PROGRAM vision
VAR
	// 系统变量，控制程序步
	State						:	CurrentState := CurrentState.Init;
	// 初始化工作步
	stepinit					:	INT := 0;
	// 载入轮廓工作步
	stepload					:	INT := 0;
	// 配方触发器
	readtrig					:	r_trig;
	// 外部触发视觉提交
	VisionTrig					:	R_TRIG;
	// 配方相关
	bReadRecipe					:	BOOL;
	// 循环/计数变量
	i							:	ULINT;
	j							:	ULINT;
	l							:	ULINT;
	m							:	DINT;
	// 视觉变量
	// 视觉系统变量
	hr							:	HRESULT;
	// 颜色
	aColorRed 					: 	TcVnVector4_LREAL := [255, 0, 0];
	aColorGreen 				: 	TcVnVector4_LREAL := [0, 255, 0];	
	aColorBlue 					: 	TcVnVector4_LREAL := [0, 20, 255];
	// 相机
	fbCamera					:	FB_VN_SimpleCameraControl;
	// 相机状态
	eState						:	ETcVnCameraState;
	// 9点标定模式相关变量
	aCircleCenter				:	TcVnPoint2_REAL;
	rCircle						:	REAL;
	aOffsetPoint				:	ARRAY[0..8] OF TcVnPoint2_REAL;
	// 标定点容器
	aSrcPoints					: 	ITcVnContainer;
	aDestPoints 				:  	ITcVnContainer;
	aOffsetPoints 				:  	ITcVnContainer;
	
	// 开启坐标变换
	bTransForm					:	BOOL; // 自动开启
	// 工作步状态信息
	// 轮廓过滤工作信息
	ContourFilterMessage		:	WSTRING;
	// 坐标变换工作信息
	GetMatrixKnMessage			:	WSTRING;
	// 错误信息
	ErrMessage					:	WSTRING;
	// 工作错误状态计时器
	ErrTon						:	ton;
	// 视觉启动延时
	VisionStartDelay			:	ton;
	// 开始工作
	bStart						:	BOOL;
	// 图片以及用于显示的绘制图像
	ipImageIn					:	ITcVnImage;// 相机输入图像
	ipImageInDisp				:	ITcVnDisplayableImage;	
	ipImageWork					:	ITcVnImage;// 工作处理图像
	ipImageWorkDisp				:	ITcVnDisplayableImage;
	ipImageRes					:	ITcVnImage;// 处理结果
	ipImageResDisp				:	ITcVnDisplayableImage;	// 结果显示窗口
	ipImageBuffer				:	ITcVnImage;// 提取坐标的时刻截取的图像
	ipImageBufferDisp			:	ITcVnDisplayableImage;	// 最近一次拍摄到的物料
	ipImageCalibration			:	ITcVnImage;// 标定坐标点记录
	ipImageCalibrationDisp		:	ITcVnDisplayableImage;
	// 轮廓提取
	// 轮廓
	ipContourList				:	ITcVnContainer;
	ipContour					:	ITcVnContainer;	
	aOffset						:	TcVnPoint;
	// 提取到的轮廓个数
	nNumberOfElements			: 	ULINT;
	// 标定模式二值化阈值
	lrCalibrationThreshold		:	LREAL := 41;
	// 采样模式二值化阈值
	lrCatchThreshold			:	LREAL := 41;
	// 二值化
	// 二值化阈值
	lrThreshold					:	LREAL := 25;
	// 结构元
	ipImageElement				:	ITcVnImage;
	// 结构元类型
	StructuralShape				:	ETcVnStructuringElementShape;
	// 结构元大小
	elementWidth				:	UDINT := 3;
	elementHeight				:	UDINT := 3;
	// 面积过滤
	fArea						:	LREAL;	// 轮廓面积
	// 手动触发视觉计算
	TrigExcute					:	BOOL := FALSE;
	// 捕获视野中的标定点坐标
	bstartGetData				:	BOOL := FALSE;
	// 刷新标定点坐标，用于标定，更新视觉中的标定点组
	bRefreshData				:	BOOL := FALSE; // 视觉9点提取
	// 手动转换
	ManualChange				:	BOOL;
	// 强制提交数据
	ForcePush					:	BOOL := FALSE;
	// 面积过滤阈值下限，用于轮廓提取
	fAreaMin					:	LREAL := 45000; // 实际面积最小值
	// 标定图形面积过滤上下限，依据标定图纸确定，需要配合专用标定纸使用
	calibrationMin				:	LREAL := 8000;
	calibrationMax				:	LREAL := 40000;
	// 坐标提取
	aCenter						:	TcVnPoint2_LREAL; // 质心坐标
	aCenterActPos				:	TcVnPoint2_LREAL; // 输出物料抓取点像素坐标
	stRectangle					:	TcVnRotatedRectangle; // 外接矩形坐标
	// 校验点
	aManualPoint				:	TcVnPoint2_LREAL;
	aRobotPoint					:	TcVnPoint2_LREAL;
	// 图片信息变量
	imageinfo					:	TcVnImageInfo;
	imageWidth					:	LREAL;	// 图片宽度（X轴方向）
	imageHeight					:	LREAL;	// 图片高度
	// 拍摄区间
	areaLength					:	LREAL := 0; // 拍摄视野的行程（可能是X或者Y）
	judgePos					:	array[0..1] of LREAL; // 用于判断物体位置的坐标
	areaBuffer					:	LREAL := 50;// 拍摄区间大小
	BeltVelo					:	LREAL := 100; // 皮带运行速度
	// 抓取点坐标
	aCenterPick					:	TcVnPoint2_LREAL; // 抓取点坐标
	// 角度
	Angle						:	LREAL;	// 与X轴（机器人坐标系）夹角（角度制）
//	fAngleTemp					:	LREAL;	// 角度临时变量
	// 缓存（用于去重）
	bmaterialBuffer1				:	DUT_material;
	// 去重坐标阈值（xy）
	xFilter						:	LREAL := 15; // X方向的偏差范围
	yFilter						:	LREAL := 15; // Y方向的偏差范围
	// 物料坐标XY偏移，用于最终调整
	xbias						:	LREAL := 0;
	ybias						:	LREAL := 0;
	// 临时字符串（用于9点标定）
	tempstr: ARRAY[0..8] OF STRING := ['0', '1', '2', '3', '4', '5', '6', '7', '8'];
	// 测量时间
	fbGetCalTime				:	Profiler;
END_VAR

CASE State OF
	CurrentState.Init:
		// 初始化模式
		Step_Init();
	
	CurrentState.Waiting:
		// 等待触发信号模式
		Step_Waiting();
		
	CurrentState.Catchmaterial:
		// 视觉系统开始工作，提取物料
		Step_Catchmaterial();
		
	CurrentState.Calibration:
		// 标定模式，配合特质的标定板，定位坐标
		Step_Calibration();
		

	CurrentState.Error:
		// 出现报错，出现各种错误
		Step_Err();
		
END_CASE

ACTION CameraStartAcquisition:
(*******************************************
切换相机状态到输出图片，复位图片检测变量
*******************************************)

// 切换相机状态
fbCamera.StartAcquisition();
// 未提取到图像
bGetImage := FALSE;
END_ACTION

ACTION ContourFilter:
(*******************************************
轮廓过滤，坐标提取
由相机自行判断中心坐标到达指定区域进行拍摄，提取相应的坐标信息
先通过面积进行粗过滤
然后通过后续的精确过滤提取到物料并做计算
*******************************************)

// 判定轮廓数量多少
IF nNumberOfElements>=1 THEN
	// 提取到至少1个轮廓
	ContourFilterMessage := "已提取到轮廓";
	
	// 重置质心坐标
	aCenter[0]:=0;
	aCenter[1]:=0;
	
	// 遍历轮廓
	FOR i:=0 TO (nNumberOfElements-1) DO
		// 提取面积
		GetContourArea();
		// 面积过滤，对不符合要求（面积特别小）的轮廓直接过滤
		IF fArea> fAreaMin THEN
			
				// 绘制轮廓
				GetAndDrawContour();			
				// 触发坐标提取，去重，信息提交
				GetMaterialMessage();
			
		END_IF		
	END_FOR

ELSE
	bVisionWarning := TRUE;
	ContourFilterMessage := "未提取到至少1个轮廓";
END_IF
END_ACTION

ACTION DrawPic:
(*******************************************
将图像绘制到可见图片，可以使用adsimage watch进行观察
*******************************************)

// 绘制图像
hr := F_VN_TransformIntoDisplayableImage(ipImageIn, ipImageInDisp, S_OK);
hr := F_VN_TransformIntoDisplayableImage(ipImageWork, ipImageWorkDisp, S_OK);		
hr := F_VN_TransformIntoDisplayableImage(ipImageRes, ipImageResDisp, S_OK);
hr := F_VN_TransformIntoDisplayableImage(ipImageBuffer, ipImageBufferDisp, S_OK);
hr := F_VN_TransformIntoDisplayableImage(ipImageCalibration, ipImageCalibrationDisp, S_OK);
END_ACTION

ACTION FindContours:
(*******************************************
轮廓提取
提取二值化后的视野中的所有轮廓
*******************************************)

// 轮廓提取
hr := F_VN_FindContoursExp(
	ipSrcImage:=ipImageWork , 
	ipContours:=ipContourList , 
	eRetrievalMode:=TCVN_CRM_EXTERNAL , 
	eApproximationMethod:=TCVN_CAM_SIMPLE , 
	aOffset:=aOffset , 
	hrPrev:=hr );
// 获取轮廓数量
hr := ipContourList.GetElementNum(nNumberOfElements);
END_ACTION

ACTION GetAndDrawContour:
(*******************************************
绘制轮廓相关信息
提取质心并绘制
提取外接矩形并绘制
提取外界矩形的几何中心并绘制
*******************************************)

// 面积满足条件
ContourFilterMessage := "已提取到面积符合的对象";
// 取得质心
hr := F_VN_ContourCenterOfMass(ipContour , aCenter, hr );
// 外接矩形
hr := F_VN_EnclosingRectangle(ipContour , stRectangle , hr );
// 在工作区域图片上绘制轮廓（绿色）
hr := F_VN_DrawContours(
		ipContours:=ipContour , 
		nContourIndex:=-1 , 
		ipDestImage:=ipImageRes , 
		aColor:=aColorGreen , 
		nThickness:=2 , 
		hrPrev:=hr );
// 在工作区域图片上绘制质心（绿色）
hr := F_VN_DrawPointExp(
		nX:=TO_UDINT(aCenter[0]), 
		nY:=TO_UDINT(aCenter[1]), 
		ipDestImage:=ipImageRes , 
		eShape:=TCVN_DS_PLUS , 
		aColor:=aColorGreen , 
		nSize:=10 , 
		nThickness:=3 , 
		eLineType:=TCVN_LT_8_CONNECTED , 
		hrPrev:=hr );
// 在工作区域图片上绘制矩形框（红色）
hr := F_VN_DrawRotatedRectangle(
		stRectangle:= stRectangle, 
		ipDestImage:= ipImageRes, 
		aColor:= aColorRed, 
		nThickness:= 3, 
		hrPrev:= hr);
// 绘制矩形的中心坐标点（红色）
hr := F_VN_DrawPointExp(
		nX:=TO_UDINT(stRectangle.aCenter[0]), 
		nY:=TO_UDINT(stRectangle.aCenter[1]), 
		ipDestImage:=ipImageRes , 
		eShape:=TCVN_DS_PLUS , 
		aColor:=aColorRed , 
		nSize:=10 , 
		nThickness:=3 , 
		eLineType:=TCVN_LT_8_CONNECTED , 
		hrPrev:=hr );
END_ACTION

ACTION GetCalibrationPoint:
(*******************************************
使用轮廓提取的方式，获取标定点坐标
*******************************************)

// 判定轮廓数量多少
IF nNumberOfElements>=1 AND bstartGetData THEN
	// 提取到至少1个轮廓
	// 遍历轮廓
	j := 0;
	FOR i:=0 TO (nNumberOfElements-1) DO
		// 提取到具体轮廓
		hr := F_VN_GetAt_ITcVnContainer(ipContourList ,ipContour , i , hr );
		// 提取轮廓面积
		hr := F_VN_ContourArea(ipContour , fArea, hr );
		// 面积过滤
		IF (fArea > calibrationMin) AND (fArea < calibrationMax) THEN;
			// 面积满足条件
			// 外接圆（圆心坐标为相对于提取区域的坐标）
			hr := F_VN_EnclosingCircle(ipPointSet:= ipContour, aCenter:= aCircleCenter, fRadius:= rCircle, hrPrev:= hr);
			hr := F_VN_EnclosingRectangle(ipContour , stRectangle , hr );
			// 绘制标定圆心
			hr := F_VN_DrawPointExp(
					nX:=TO_UDINT(aCircleCenter[0]), 
					nY:=TO_UDINT(aCircleCenter[1]), 
					ipDestImage:=ipImageRes , 
					eShape:=TCVN_DS_PLUS , 
					aColor:=aColorGreen , 
					nSize:=10 , 
					nThickness:=3 , 
					eLineType:=TCVN_LT_8_CONNECTED , 
					hrPrev:=hr );
			// 提取到的坐标注入数组
			IF j <= 8 THEN
				// 绘制点号
				hr := F_VN_PutTextExp(
					sText:= tempstr[j], 
					ipDestImage:= ipImageRes, 
					nX:= TO_UDINT(aCircleCenter[0]+25), 
					nY:= TO_UDINT(aCircleCenter[1] + 25), 
					eFontType:= ETcVnFontType.TCVN_FT_HERSHEY_PLAIN, 
					fFontScale:= 10, 
					aColor:= aColorRed, 
					nThickness:= 4, 
					eLineType:= 4, 
					bBottomLeftOrigin:= FALSE, 
					hrPrev:= hr);
				// 更新视觉矩阵数组
				IF bRefreshData THEN
					aSrcPoint[j][0] := aCircleCenter[0];
					aSrcPoint[j][1]	:= aCircleCenter[1];
				END_IF
				j := j+ 1;
			END_IF
			IF bRefreshData THEN
				hr := F_VN_CopyImageRegion(
					ipSrcImage:= ipImageRes, 
					nX:= 0, 
					nY:= 0, 
					nWidth:= imageinfo.nWidth, 
					nHeight:= imageinfo.nHeight, 
					ipDestImage:= ipImageCalibration, 
					hrPrev:= hr);
			END_IF
		END_IF
	END_FOR
END_IF
END_ACTION

ACTION GetContourArea:
(*******************************************
轮廓面积提取
对于轮廓进行面积计算
*******************************************)

// 有轮廓
bVisionWarning := FALSE;
// 提取到具体轮廓
hr := F_VN_GetAt_ITcVnContainer(ipContourList ,ipContour , i , hr );
// 提取轮廓面积
hr := F_VN_ContourArea(ipContour , fArea, hr );
END_ACTION

ACTION GetdMaterial:
(*******************************************
数据注入结构体
*******************************************)

// 注入机器人结构体
dMaterial.bMaterial := TRUE;
// 机器人需要旋转的角度为机器人坐标正向90度
IF Angle < 90 THEN
	dMaterial.lrAngle :=  (Angle);
ELSE
	dMaterial.lrAngle := -(90 - Angle);
END_IF
//dMaterial.lrAngle := Angle;
// 提取点坐标注入
dMaterial.lrCenterX := aCenterActPos[0] + xbias;// 坐标偏置
dMaterial.lrCenterY := aCenterActPos[1] + ybias;
// 输出面积
dMaterial.lrArea := fArea;	
// 拍摄图片的时间（获取系统时间求得）
dMaterial.lrPhotoTime := ULINT_TO_LREAL(F_GetSystemTime()) / 10000000;
dMaterial.lrPhotoBeltPos:=BeltAxis.NcToPlc.ActPos;
END_ACTION

ACTION GetImageWH:
(*******************************************
读取图片信息，主要是获取宽度值
*******************************************)

// 读取相机输入图像信息
hr := F_VN_GetImageInfo(ipImage:= ipImageIn, stImageInfo:= imageinfo, hrPrev:= hr);

// 将信息提取到指定变量
imageWidth := TO_LREAL(imageinfo.nWidth);
imageHeight := TO_LREAL(imageinfo.nHeight);
END_ACTION

ACTION GetMaterialMessage:
(*******************************************
拍摄
计算指定区间
判断外接矩形的中心坐标是否达到指定区域
如果到达指定区域，则对物料做后续计算以及坐标提取
*******************************************)


// 手动触发器，如果触发，则强制拍摄
VisionTrig(CLK:= TrigExcute, Q=> );
// 使用X判断/Y判断，皮带的X方向与相机的X方向/Y方向重合，建议不要使用，需要修改后续的逻辑
	areaLength := imageHeight / 2;
	judgePos[0] := stRectangle.aCenter[1];
	judgePos[1] := stRectangle.aCenter[0];
// 判断外接矩形的中心点是否在指定区域或强制推送
IF (judgePos[0] > areaLength - areaBuffer) AND (judgePos[0] < areaLength + areaBuffer) AND (judgePos[1] > 200) AND (judgePos[1] < (imageWidth - 200)) 
	OR VisionTrig.Q OR ForcePush THEN
	// 通过矩形的角度求得实际物体的部署角度
	Angle := TO_LREAL(stRectangle.fAngle);
	
	// 提取点坐标，提取点坐标为质心坐标
		aCenterPick[0] := aCenter[0];
		aCenterPick[1] := aCenter[1];
		
	
	
	// 绘制提取点
	hr := F_VN_DrawPointExp(
		nX:=TO_UDINT(aCenterPick[0]), 
		nY:=TO_UDINT(aCenterPick[1]), 
		ipDestImage:=ipImageRes , 
		eShape:=TCVN_DS_PLUS , 
		aColor:=aColorBlue , 
		nSize:=10 , 
		nThickness:=3 , 
		eLineType:=TCVN_LT_8_CONNECTED , 
		hrPrev:=hr );
		
	// 结果注入队列
	PushbMaterial();
END_IF
END_ACTION

ACTION GetTransformationMatrixKn:
(*******************************************
生成变换矩阵
将变换矩阵用的点位（视觉坐标系9点，机器人坐标系9点），分别注入container
通过2个container求解变换矩阵
*******************************************)

// 坐标变换
FOR j := 0 TO 8 BY 1 DO
	// 机器人坐标系标定时需要减去皮带偏移，相机不在机器人正下方
	aOffsetPoint[j][0] := aDestPoint[j][0] - lrBeltOffset;
	aOffsetPoint[j][1] := aDestPoint[j][1];
END_FOR

// 生成变换点集
hr := F_VN_CreateContainerFromArray(
	pData:= ADR(aSrcPoint), 
	ipContainer:= aSrcPoints, 
	nTypeGuid:= ContainerType_Vector_TcVnPoint2_REAL, 
	nElementNum:= 9, 
	hrPrev:= 0);// 视觉像素点集
hr := F_VN_CreateContainerFromArray(
	pData:= ADR(aOffsetPoint), 
	ipContainer:= aOffsetPoints, 
	nTypeGuid:= ContainerType_Vector_TcVnPoint2_REAL, 
	nElementNum:= 9, 
	hrPrev:= 0);// 机器人坐标系点集

// 判断点集合是否有效（如果没有成功上载配方，点集可能是无效的，将会触发pagefault）
IF (aSrcPoints <> 0) AND (aOffsetPoints <> 0) THEN
	// 获取变换矩阵
	hr := F_VN_Homography(aSrcPoints, aOffsetPoints, aTransformationMatrix, 0);
	// 坐标变换矩阵求解成功，开启坐标变换
	bTransForm := TRUE;
	GetMatrixKnMessage := "";
ELSE
	// 点集合无效，报错
	bVisionWarning := TRUE;
	bTransForm := FALSE;
	GetMatrixKnMessage := "无效坐标点或变换矩阵";
END_IF


// 释放
FW_SafeRelease(ADR(aSrcPoints));
FW_SafeRelease(ADR(aDestPoints));
END_ACTION

ACTION Halt:
(*******************************************
如果触发了停止信号，就将状态机切换到Waiting状态
*******************************************)

// 触发停止动作
IF VisionHalt THEN
	// 切换到等待状态
	State := CurrentState.Waiting;
	// 对停止信号进行复位操作
	VisionHalt := FALSE;
END_IF
END_ACTION

ACTION Pretreatment:
(*******************************************
预处理
将输入图像转换为三通道图像注入结果图像（方便后续绘制轮廓等）
将输入图像进行二值化，注入工作图像，用于后续计算
*******************************************)

// 单通道变为三通道(RGB)注入结果图像
hr := F_VN_ConvertColorSpace(ipImageIn ,ipImageRes , TCVN_CST_GRAY_TO_RGB , hr );
// 二值化
hr := F_VN_Threshold(
	ipSrcImage:=ipImageIn , 
	ipDestImage:=ipImageWork , 
	fThreshold:=lrThreshold , 
	fMaxValue:=255 , 
	eThresholdType:=TCVN_TT_BINARY , 
	hrPrev:=hr );
END_ACTION

ACTION PushbMaterial:
(*******************************************
坐标变换，去重，提交数据
去重的思路为，物料X坐标以及Y坐标是否一致，一致的话就认为是同一个
对于目前的情况，X坐标还需要减去两次拍摄之间皮带的偏移量
*******************************************)

IF bTransForm THEN
	// 将中心坐标使用变换矩阵转换为机器人坐标系
	hr := F_VN_WarpPerspective_Point(aCenterPick ,aCenterActPos , aTransformationMatrix , hr );
	// 本次拍摄结果坐标与上一次拍摄结果坐标比对进行去重计算，计算xy坐标是否相近，相近则判断为同一个，不做提交
	IF (ABS(bMaterialBuffer1.lrCenterY - aCenterActPos[1]) > YFilter) OR 
	(ABS(ABS(bMaterialBuffer1.lrCenterX - aCenterActPos[0]) - ABS(bMaterialBuffer1.lrPhotoBeltPos - beltAxis.NcToPlc.ActPos)) > YFilter) THEN
			// 注入结构体
			GetdMaterial();
			
			// 绘制提取点
			hr := F_VN_DrawPointExp(
					nX:=TO_UDINT(aCenterPick[0]), 
					nY:=TO_UDINT(aCenterPick[1]), 
					ipDestImage:=ipImageRes , 
					eShape:=TCVN_DS_PLUS , 
					aColor:=aColorBlue , 
					nSize:=10 , 
					nThickness:=3 , 
					eLineType:=TCVN_LT_8_CONNECTED , 
					hrPrev:=hr );
			
			
				// 压入队列
				gfbPushPopStack(ArrayStmaterial:=gArrayStmaterial , PushStmaterial:=dmaterial , PopStmaterial=> , busy=>gbPushPopBusy );
				gfbPushPopStack.PushStack();
				fbGetCalTime(START:= FALSE, RESET:= FALSE, BUSY=> , DATA=> );			
			// 将最后一个写入队列的dmaterial设置为比较对象
			MEMCPY(destAddr:= ADR(bMaterialBuffer1), srcAddr:= ADR(dMaterial), n:= SIZEOF(bMaterialBuffer1));
		
			// 记录拍摄瞬间的时刻的图像
			hr := F_VN_CopyImage(ipSrcImage:= ipImageRes, ipDestImage:= ipImageBuffer, hrPrev:= hr);
	END_IF
END_IF
END_ACTION

ACTION RecipeSaveAndRead:
(*******************************************
配方操作
通过设置好的配方名称，对配方进行读
由于配方主要用于矩阵的保存以及读取，而TwinCAT的配方无法直接保存TcVnPoint2_LREAL型的视觉点变量，因此要先转换为普通的二维数组点
*******************************************)


// 读取配方触发器
readtrig(CLK:= bReadRecipe , Q=> );

// 触发器触发
IF  readtrig.Q THEN
		// 触发读取配方，将配方点数组读取后，写入视觉矩阵
	FOR l := 0 TO 8 BY 1 DO
		aSrcPoint[l][0] := srcpoint[l, 0];
		aSrcPoint[l][1] := srcpoint[l, 1];
		aDestPoint[l][0] := destpoint[l, 0];
		aDestPoint[l][1] := destpoint[l, 1];
	END_FOR
END_IF
END_ACTION

ACTION Release:
(*******************************************
释放内存
*******************************************)

FW_SafeRelease(ADR(ipContourList));
FW_SafeRelease(ADR(ipContour));
END_ACTION

ACTION Step_Calibration:
(*******************************************
标定模式
用于更新参数
将视觉坐标系以及机器人坐标系进行对应
*******************************************)

// 读取相机状态
eState := fbCamera.GetState();

// 相机停止状态监控
Halt();

// 根据状态进行操作
CASE eState OF
// 相机初始化
TCVN_CS_INITIAL,TCVN_CS_OPENING,TCVN_CS_OPENED,TCVN_CS_STARTACQUISITION:
	// 切换相机状态
	CameraStartAcquisition();

TCVN_CS_ACQUIRING:
	// 复位错误计时器
	ErrTon.IN := FALSE;
	// 获取图片
	hr := fbCamera.GetCurrentImage(ipImageIn);
	// 图片采样成功
	IF tc3_module.SUCCEEDED(hr) AND ipImageIn <> 0 THEN
		// 图片提取成功
		bGetImage := TRUE;
		
		// 修改二值化阈值
		lrThreshold := lrCalibrationThreshold;
		
		// 预处理
		Pretreatment();
		
		// 像素取反（标定用的纸为白底黑色圆，需要前景背景替换）
		hr := F_VN_BitwiseNotImage(ipSrcImage:= ipImageWork, ipDestImage:= ipImageWork, hrPrev:= hr);
		// 闭运算
		hr := F_VN_CreateStructuringElement(
			ipStructuringElement:= ipImageElement, 
			eShape:= StructuralShape, 
			nWidth:= elementWidth, 
			nHeight:= elementHeight, 
			hrPrev:= hr);
		hr := F_VN_MorphologicalOperator(
			ipSrcImage:= ipImageWork, 
			ipDestImage:= ipImageWork, 
			eOperator:= TCVN_MO_CLOSING, 
			ipStructuringElement:= ipImageElement, 
			hrPrev:= hr);
		
		// 轮廓提取
		FindContours();
		
		// 获取坐标点
		GetCalibrationPoint();
		
		// 更新坐标变换矩阵
		GetTransformationMatrixKn();
		
		// 校验标定
		IF ManualChange THEN
			// 手动转换，将视觉坐标转换成机器人坐标
			hr := F_VN_WarpPerspective_Point(aManualPoint ,aRobotPoint , aTransformationMatrix , hr );
		END_IF
		
		// 坐标保存(暂时未研究如何配合hmi的recipe)
	//	RecipeSaveAndRead();
		
		// 绘制图像
		DrawPic();

	ELSE
		// 未提取到图像
		bGetImage := FALSE;
	END_IF

Tc3_Vision.TCVN_CS_ERROR:
	// 执行报错动作
	VisionError();
END_CASE
END_ACTION

ACTION Step_Catchmaterial:
(*******************************************
拍摄
正常工作状态
相机无限制拍摄图片，根据拍摄出的图片进行相应的坐标计算，并返还结果
*******************************************)

// 读取相机状态
eState := fbCamera.GetState();

// 相机停止状态监控
Halt();

// 根据状态进行操作
CASE eState OF
// 相机初始化
TCVN_CS_INITIAL,TCVN_CS_OPENING,TCVN_CS_OPENED,TCVN_CS_STARTACQUISITION:
	// 切换相机状态
	CameraStartAcquisition();
	
TCVN_CS_ACQUIRING:
	// 复位错误计时器
	ErrTon.IN := FALSE;
	// 获取图片
	hr := fbCamera.GetCurrentImage(ipImageIn);
	// 图片采样成功
	IF tc3_module.SUCCEEDED(hr) AND ipImageIn <> 0 THEN
		// 图片提取成功
		bGetImage := TRUE;
		
		// 计算时间
//		fbGetCalTime(START:= FALSE, RESET:= TRUE, BUSY=> , DATA=> );
//		fbGetCalTime(START:= TRUE, RESET:= FALSE, BUSY=> , DATA=> );
		// 重新设置二值化阈值到拍摄模式
		lrThreshold := lrCatchThreshold;
		
		
		// 预处理
		Pretreatment();

		// 轮廓提取
		FindContours();
		
		// 由相机自行判断中心坐标到达指定区域进行拍摄，提取相应的坐标信息
		ContourFilter();
		
		// 释放
		Release();
		
		// 绘制图像
		DrawPic();
		
	ELSE
		// 未提取到图像
		bGetImage := FALSE;
	END_IF
	
Tc3_Vision.TCVN_CS_ERROR:
	// 执行报错动作
	VisionError();
END_CASE
END_ACTION

ACTION Step_Err:
(*******************************************
报错状态，输出错误标志位以及报警信息
*******************************************)

bVisionErr := TRUE;
VisionErrMessage := Tc2_Standard.WCONCAT("视觉系统报错，报错信息：", Errmessage);
END_ACTION

ACTION Step_Init:
(*******************************************
初始步
对参数以及文件目录初始化
生成变换矩阵
检测视觉是否成功采集到图像
获取图像长宽等信息
如果一切正常，则自动切换进入等待模式
*******************************************)

CASE stepinit OF
	
		
	
	
	0:// 上载配方
		// 触发配方读动作
		//bReadRecipe := TRUE;
		// 配方程序
		RecipeSaveAndRead();
		stepinit := 40;
		
	40:// 复位配方程序
		RecipeSaveAndRead();
		bReadRecipe := FALSE;
		stepinit := 50;
		
	50:// 数据准备
		// 更新变换矩阵
		GetTransformationMatrixKn();
		// 复位错误状态
		bVisionErr := FALSE;
		Errmessage := "";
		ErrTon.IN := FALSE;
		stepinit := 60;
		
	60:// 检查是否拍摄到图像
		// 读取相机状态
		eState := fbCamera.GetState();
		
		// 根据状态进行操作
		CASE eState OF
			// 相机初始化
			TCVN_CS_INITIAL,TCVN_CS_OPENING,TCVN_CS_OPENED,TCVN_CS_STARTACQUISITION:
				// 切换相机状态
				CameraStartAcquisition();
				
			// 开始获取照片
			TCVN_CS_ACQUIRING:
				// 复位错误计时器
				ErrTon.IN := FALSE;
				// 获取图片
				hr := fbCamera.GetCurrentImage(ipImageIn);
				// 图片采样成功
				IF tc3_module.SUCCEEDED(hr) AND ipImageIn <> 0 THEN
					// 提取到图像成功
					bGetImage := TRUE;
					// 获取视野的长宽
					GetImageWH();
					// 坐标变换正常激活，图片宽高提取成功
					IF bTransForm AND (imageHeight <> 0) AND (imageHeight <> 0) THEN
						// 延时，告知视觉已经就绪
						VisionStartDelay(IN:= bStart, PT:= T#1S, Q=> VisionReady, ET=> );
						bStart := TRUE;
						// 切换到等待模式
						IF VisionReady THEN
							// 视觉状态通过，切换到下一步
							State := CurrentState.Waiting;
							bStart := FALSE;
						END_IF	
					END_IF
					// 绘制图像
					DrawPic();
				ELSE
					// 未提取到图像
					bGetImage := FALSE;
				END_IF
				
			Tc3_Vision.TCVN_CS_ERROR:
					// 执行报错动作
					VisionError();
		END_CASE
END_CASE
END_ACTION

ACTION Step_Waiting:
(*******************************************
等待模式
等待视觉系统开启信号
开启信号可能由主控程序提供，或者是由调试界面输出
*******************************************)

// 如果允许开启视觉系统
IF VisionStartPush THEN
	// 切换到推送图片
	State := CurrentState.Catchmaterial;
	// 对开启信号进行复位操作
	VisionStartPush := FALSE;
END_IF
END_ACTION

ACTION VisionError:
(*******************************************
相机出现报错，检测报错能否复位，无法复位则直接切换整个程序步到错误状态
*******************************************)

// 复位相机
fbCamera.Reset();
// 未提取到图像
bGetImage := FALSE;
// 错误计时
ErrTon(IN:= TRUE, PT:= T#10S, Q=> , ET=> );
IF ErrTon.Q THEN
	// 切换视觉程序到错误异常模式
	State := CurrentState.Error;
	// 输出相机错误信息
	Errmessage := "相机工作状态异常";
END_IF
END_ACTION

END_PROGRAM
